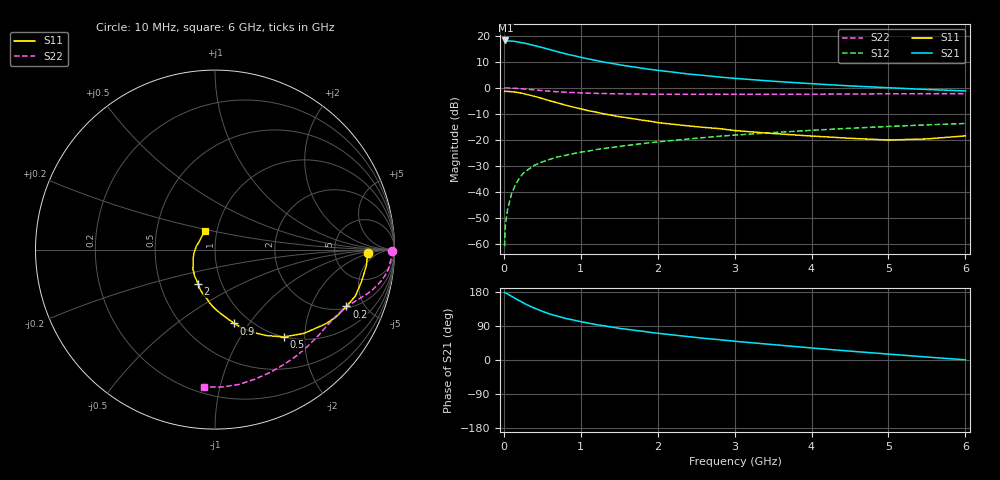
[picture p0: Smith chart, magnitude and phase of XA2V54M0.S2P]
! SIEMENS Discrete & RF Semiconductors
! BFY180
! Si NPN RF Bipolar Junction Transistor in MICRO-X
! VCE = 2.5 V  IC = 4 mA
! Common Emitter S-Parameters:  May  1997
# GHz  S  MA  R  50
!  f  S11  S21  S12  S22
! GHz  MAG  ANG  MAG  ANG  MAG  ANG  MAG  ANG
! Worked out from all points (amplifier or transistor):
!   36 points, 10 MHz to 6 GHz, reference 50 ohm
!   highest |S21| = 18.1 dB at 20 MHz (marker M1)
!   |S21| within 3 dB of that: start of sweep to 533.9 MHz
!   unconditionally stable (mu >= 1): 1.321 GHz to end of sweep
!   at 250 MHz: K = 0.28, MSG = 25.1 dB, |S12| = -33.0 dB
!   at 1.4 GHz: K = 1.03, MAG = 15.1 dB, |S12| = -23.0 dB
!   at 6 GHz: K = 1.14, MAG = 4.0 dB, |S12| = -13.8 dB
!   S11 on the Smith chart (normalised r, x): 10 MHz: 12, -2; 200 MHz: 2.11, -3.68; 500 MHz: 1.00, -1.58; 900 MHz: 0.85, -0.85; 2 GHz: 0.77, -0.31; 6 GHz: 0.88, +0.19
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0.01  0.8499 -1.2  7.927 178.5  0.0009 94.0  0.9863 -0.3
0.02  0.8494 -2.5  8.079 177.3  0.0023 94.0  0.9872 -0.8
0.05  0.8486 -5.8  7.897 174.1  0.0047 83.9  0.9871 -2.2
0.1  0.8363 -12.1  7.844 168.2  0.0091 85.7  0.9777 -4.3
0.15  0.8236 -18.3  7.715 162.1  0.0135 81.3  0.973 -6.4
0.2  0.7975 -23.4  7.478 156.6  0.0181 77.0  0.9605 -8.3
0.3  0.7398 -34.2  7.004 145.7  0.0257 70.1  0.9318 -11.7
0.4  0.6808 -43.3  6.43 136.7  0.0324 67.0  0.9051 -14.4
0.5  0.6192 -51.8  5.901 128.5  0.0374 63.4  0.8782 -16.6
0.6  0.5589 -59.0  5.381 121.0  0.0421 60.8  0.8539 -18.4
0.7  0.5095 -65.1  4.912 115.6  0.0468 58.8  0.8342 -20.1
0.8  0.4622 -71.0  4.479 109.9  0.05 57.5  0.8175 -21.5
0.9  0.4252 -75.4  4.155 105.6  0.0539 56.2  0.8043 -22.9
1.1  0.3611 -84.3  3.563 97.3  0.0605 54.9  0.7852 -25.5
1.5  0.2768 -99.5  2.764 83.7  0.0744 52.7  0.7623 -30.8
2  0.2132 -116.3  2.154 70.6  0.0907 50.1  0.7505 -37.8
2.2  0.1982 -121.4  1.993 66.1  0.097 49.1  0.7483 -40.6
2.8  0.1634 -139.0  1.602 53.6  0.1165 45.4  0.7451 -49.0
3.5  0.1314 -158.0  1.33 40.6  0.1371 40.8  0.7464 -58.6
4.5  0.1066 171.2  1.081 23.4  0.166 33.3  0.755 -72.6
5.5  0.1036 134.9  0.923 7.8  0.1929 25.5  0.7668 -87.3
6  0.1186 117.2  0.866 0.5  0.2052 21.2  0.7675 -94.7
